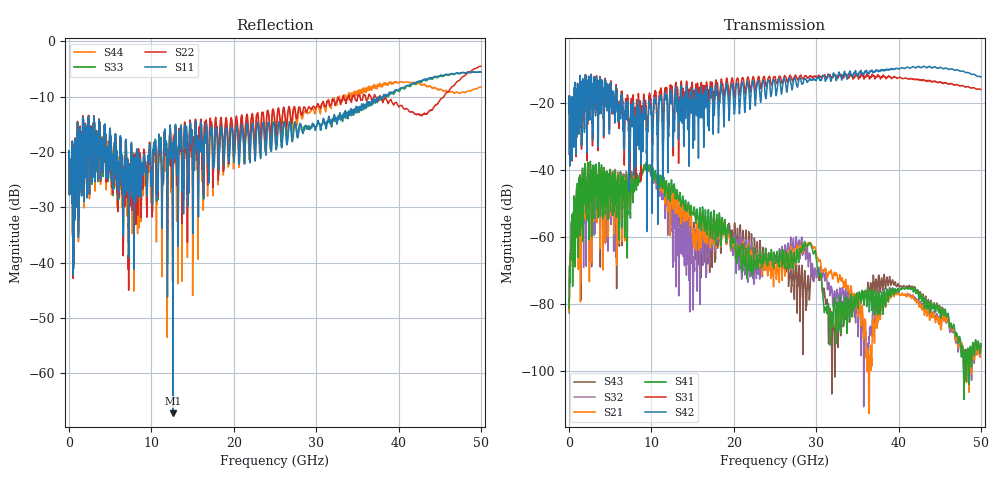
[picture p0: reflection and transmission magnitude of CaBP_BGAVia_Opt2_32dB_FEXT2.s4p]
!* Samtec Inc. NovaRay Examax Flyover System  *
!*  REV DATE  = 08/08/18  *
!*  TYPE  = TOUCHSTONE  *
!*  PORTS  = 4 port  *
!*  UNITS  = GHz  *
!*  DATA RANGE = DC  to 50 GHz; 10 MHz Step  *
!*  PARAMETER  = S  *
!*  FORMAT  = Real-Imaginary  *
!*  REFERENCE  = 50 ohms  *
!*  SOURCE  = HFSS  *
!*  VALIDATED  = No  *
!*  MANUFACTURER = SAMTEC  *
!*  INTERCONNECT = NVAx to EBCx to EBCx to NVAx  *
!*  [Full Channel NVAx to EBCx to EBCx to NVAx  with PCB Trace and BGA Via]  *
!*  BOUNDARY A  = Silicon BGA Ball Pad  *
!*  BOUNDARY B  = Silicon BGA Ball Pad  *
!*  NVAx (end a) ->>- (end b) NVAx  *
!*  Port 01 ->>- Port 02  *
!*  Port 03 ->>- Port 04  *
!***************************** CHANNEL MODEL ******************************************
# GHz S RI R 50
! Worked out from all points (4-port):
!   5000 points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, 10 MHz to 50 GHz, reference 50 ohm
!   strongest paths, dB at 10 MHz, 12.51 GHz, 25.01 GHz, 37.51 GHz, 50 GHz:
!     S42: -23.1, -17.6, -14.4, -10.6, -12.3
!     S31: -23.1, -15.2, -12.2, -11.7, -16.1
!     S41: -81.5, -45.7, -65.7, -81.9, -92.1
!     S21: -82.3, -49.4, -69.3, -83.5, -93.2
!     S32: -82.8, -56.5, -67.0, -80.2, -93.1
!     S43: -81.8, -50.1, -67.1, -74.7, -92.0
!   lowest |S11| = -67.2 dB at 12.6 GHz (marker M1), VSWR 1.00, Z = 50 + j0.0147 ohm
!   |S11| at or under -10 dB: start of sweep to 37.74 GHz; 37.74 GHz to 38.13 GHz (385.5 MHz wide, 1.02 % of centre); 38.51568 GHz to 38.54961 GHz (33.93 MHz wide, 0.0881 % of centre)
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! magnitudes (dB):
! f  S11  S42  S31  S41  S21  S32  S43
! 10 MHz  -21.6  -23.1  -23.1  -81.5  -82.3  -82.8  -81.8
! 1.75 GHz  -15.0  -13.3  -13.1  -45.6  -48.2  -51.6  -48.3
! 12.6 GHz  -67.2  -24.8  -21.8  -46.7  -51.4  -63.5  -52.5
! 22.11 GHz  -16.7  -16.4  -15.4  -67.2  -65.5  -67.2  -63.9
! 29.26 GHz  -15.9  -12.9  -11.9  -61.9  -61.8  -65.5  -75.4
! 31.14 GHz  -15.0  -13.6  -12.6  -81.3  -69.6  -71.4  -79.3
! 50 GHz  -5.5  -12.3  -16.1  -92.1  -93.2  -93.1  -92.0
